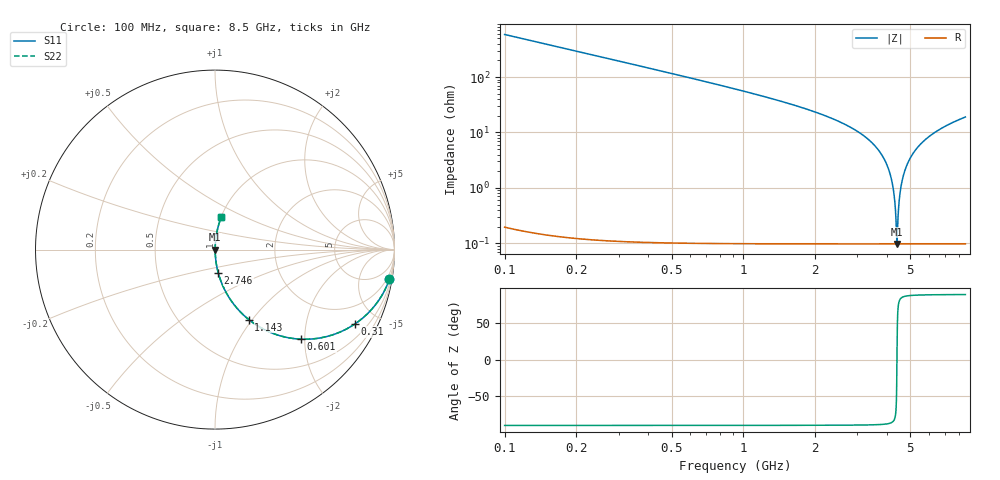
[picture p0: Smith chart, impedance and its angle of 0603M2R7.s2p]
! Created Wed Apr 18 15:30:14 2012
# hz S ma R 50
! 2 Port Network Data from SP1.SP block
! freq  magS11  angS11  magS21  angS21  magS12  angS12  magS22  angS22
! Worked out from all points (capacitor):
!   8401 points, 100 MHz to 8.5 GHz, reference 50 ohm
!   read as one part in series: C = 2.7 pF near 142 MHz
!   lowest |Z| = 97.1 mohm at 4.394 GHz (marker M1)
!   series resonance near 4.394 GHz, so ESL is about 490 pH
!   S11 on the Smith chart (normalised r, x): 100 MHz: 1, -12; 310 MHz: 1.00, -3.78; 601 MHz: 1.00, -1.92; 1.143 GHz: 1.00, -0.96; 2.746 GHz: 1.00, -0.26; 8.5 GHz: 1.00, +0.38
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1e8  0.9858 -9.6  0.1673 80.3  0.1673 80.3  0.9858 -9.6
3.1e8  0.8839 -27.9  0.4672 62.1  0.4672 62.1  0.8839 -27.9
6.01e8  0.6931 -46.1  0.7201 43.9  0.7201 43.9  0.6931 -46.1
1.143e9  0.433 -64.2  0.9005 25.7  0.9005 25.7  0.433 -64.2
1.5e9  0.3277 -70.7  0.9439 19.1  0.9439 19.1  0.3277 -70.7
2.746e9  0.1296 -82.1  0.9906 7.4  0.9906 7.4  0.1296 -82.1
2.9e9  0.1139 -83.0  0.9925 6.5  0.9925 6.5  0.1139 -83.0
3.493e9  0.06194 -85.6  0.9971 3.6  0.9971 3.6  0.06194 -85.6
3.895e9  0.03238 -86.4  0.9985 1.9  0.9985 1.9  0.03238 -86.4
4.153e9  0.01515 -85.5  0.9989 0.9  0.9989 0.9  0.01515 -85.5
4.238e9  0.009726 -83.7  0.999 0.6  0.999 0.6  0.009726 -83.7
4.3e9  0.005862 -80.1  0.999 0.3  0.999 0.3  0.005862 -80.1
4.367e9  0.001901 -59.2  0.999 0.1  0.999 0.1  0.001901 -59.2
4.394e9  0.0009703 1.1  0.999 -0.0  0.999 -0.0  0.0009703 1.1
4.418e9  0.001769 56.7  0.999 -0.1  0.999 -0.1  0.001769 56.7
4.472e9  0.004836 78.2  0.999 -0.3  0.999 -0.3  0.004836 78.2
4.528e9  0.008134 82.7  0.999 -0.5  0.999 -0.5  0.008134 82.7
4.728e9  0.0197 86.1  0.9988 -1.1  0.9988 -1.1  0.0197 86.1
5.105e9  0.04038 86.3  0.9982 -2.3  0.9982 -2.3  0.04038 86.3
5.7e9  0.07045 85.2  0.9965 -4.0  0.9965 -4.0  0.07045 85.2
7.1e9  0.1326 82.0  0.9902 -7.6  0.9902 -7.6  0.1326 82.0
8.5e9  0.187 78.9  0.9814 -10.8  0.9814 -10.8  0.187 78.9
